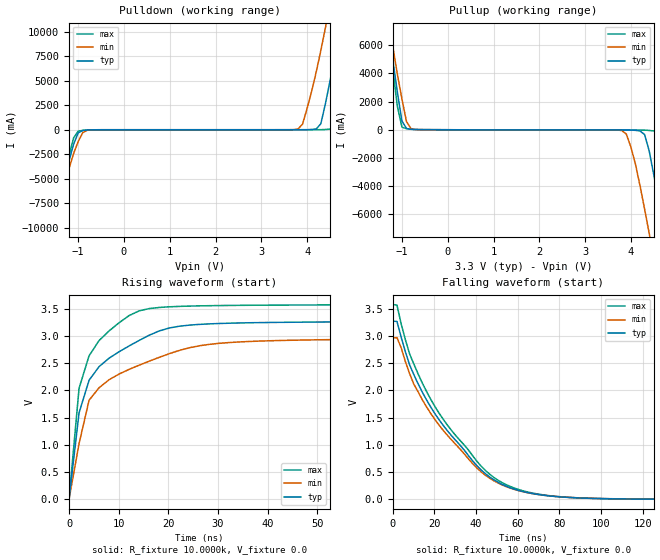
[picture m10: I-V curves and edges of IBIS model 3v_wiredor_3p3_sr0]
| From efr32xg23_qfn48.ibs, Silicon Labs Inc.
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|   Model 3v_wiredor_3p3_sr0
[Model]  3v_wiredor_3p3_sr0
Model_type Output
Polarity   Non-Inverting
Enable   Active-Low
C_comp   1.6300pF   1.4000pF   2.7000pF
[Temperature Range]   25.0000   0.1250k   -40.0000
[Pullup Reference]   3.3000V   3.0000V   3.6000V
[Pulldown Reference]   0.0V   0.0V   0.0V
[POWER Clamp Reference]   3.3000V   3.0000V   3.6000V
[GND Clamp Reference]   0.0V   0.0V   0.0V
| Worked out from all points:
|   slope of the pullup table from 0 to 0.495 V, typ, clamps not added: 103 ohm
|   rising waveform, R_fixture 10.0000k, V_fixture 0.0: 20-80 % time 7.68ns typ, 10.6ns min, 4.95ns max; typ from 0 V to 3.27 V
|   falling waveform, R_fixture 10.0000k, V_fixture 0.0: 20-80 % time 32.7ns typ, 32.4ns min, 33.5ns max; typ from 3.27 V to 0.001 V
[Pulldown]
|Voltage   I(typ)   I(min)   I(max)
-3.3V     -36.82A    -34.37A    -38.92A
-1.6V     -10.63A    -10.8A     -10.59A
-1V       -326.3mA   -1.208A    -136.6mA
-700mV    -7.474mA   -9.083mA   -8.231mA
3.8V      591.9uA    67.26mA    3.714nA
4V        6.191mA    2.175A     19.25uA
4.3V      614.4mA    8.098A     6.516mA
4.4V      2.66A      10.42A     23.07mA
4.6V      7.505A     15.17A     173.2mA
4.7V      10.17A     17.48A     1.662A
5V        18.27A     24.04A     10.12A
6.6V      55.71A     55.21A     53.88A
[Pullup]
|Voltage   I(typ)   I(min)   I(max)
-3.3V     55.71A     49.41A     61.66A
-1.3V     7.509A     8.099A     7.144A
-1.1V     2.665A     3.945A     1.669A
-900mV    88.8mA     574.5mA    74.57mA
3.8V      -14.96mA   -56.37mA   -19.92mA
4V        -21.75mA   -1.218A    -20.01mA
4.3V      -340.6mA   -5.62A     -28.27mA
4.4V      -1.497A    -7.339A    -48.76mA
4.6V      -4.988A    -10.81A    -156.7mA
4.7V      -6.861A    -12.5A     -857.2mA
5.1V      -14.26A    -18.6A     -8.605A
6.6V      -36.84A    -38.17A    -34.32A
[Ramp]
| variable   typ   min   max
dV/dt_r  1.9613/7.6782n   1.7760/10.5601n   2.1440/4.9539n
dV/dt_f  8.5324u/2.6415p   62.7070u/31.0965n   8.5871u/1.4522p
R_load = 10.0000k
[Rising Waveform]
R_fixture= 10.0000k
V_fixture= 0.0
V_fixture_min= 0.0
V_fixture_max= 0.0
|time   V(typ)   V(min)   V(max)
0s        13.25uV    93.35uV    24.31uV
2.02ns    1.589V     1.022V     2.038V
4.04ns    2.186V     1.818V     2.634V
6.061ns   2.435V     2.049V     2.914V
10.1ns    2.708V     2.299V     3.241V
16.16ns   3.011V     2.535V     3.499V
20.2ns    3.143V     2.672V     3.531V
26.26ns   3.209V     2.817V     3.548V
42.42ns   3.246V     2.913V     3.562V
200ns     3.269V     2.96V      3.573V
[Falling Waveform]
R_fixture= 10.0000k
V_fixture= 0.0
V_fixture_min= 0.0
V_fixture_max= 0.0
|time   V(typ)   V(min)   V(max)
0s        3.269V     2.962V     3.574V
2.02ns    3.262V     2.965V     3.561V
6.061ns   2.706V     2.525V     2.927V
10.1ns    2.288V     2.113V     2.483V
22.22ns   1.46V      1.361V     1.581V
42.42ns   538.6mV    504.4mV    609mV
54.55ns   240.9mV    232mV      267.7mV
68.69ns   95.81mV    95.43mV    104mV
88.89ns   26.98mV    28.43mV    28.14mV
200ns     958.9uV    1.275mV    801.6uV
